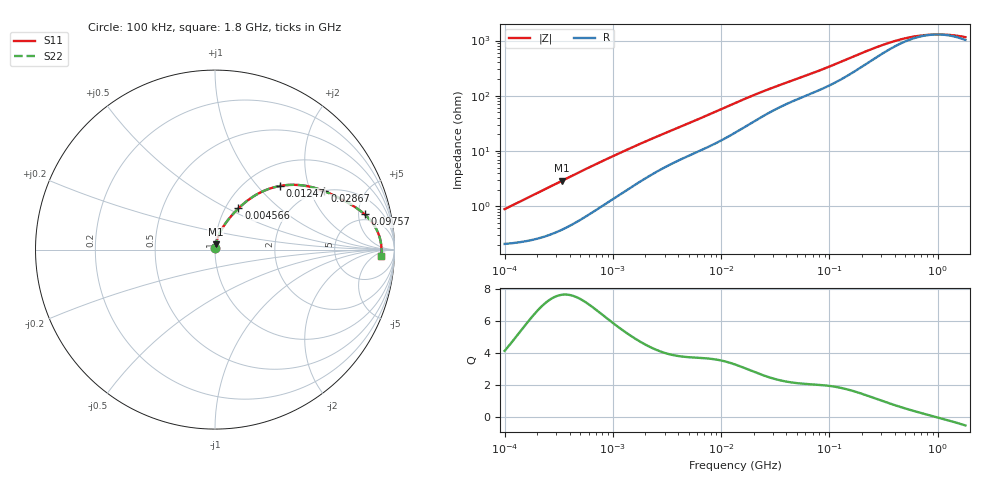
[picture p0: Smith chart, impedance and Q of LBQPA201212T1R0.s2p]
! LBQPA201212T1R0  S-PARAMETER MODEL  ( General Type )
! Model Generated by TAIYO YUDEN Corporation (http://www.ty-top.com)
! Version 1.0
! TAIYO YUDEN Control No. 191025NI43SB-FBB
! Copyright(c) 2019 TAIYO YUDEN CO.,LTD. All Rights Reserved.
! Product Description (link to TY-COMPAS)
! https://ds.yuden.co.jp/TYCOMPAS/or/detail?pn=LBQPA201212T1R0M&u=M
! Products Name : Inductors
! Characteristics :
!  Inductance : 1.0 uH , SRF(min) : 100 MHz , DC Resistance(max) : 0.247 Ohm
!  Rated Current : Saturation :700 mA , Temp Rise : 640 mA (20 degC)
!  Case Size : 2.0 x 1.25 / 0.079 x 0.049 [mm/inch] , Thickness : 1.25 / 0.049 [mm/inch]
!  (Conditions: Temperature = 25 degC , DC Bias Current/Voltage = 0A / 0V)
! External Node Assignments :
!  1  o---GGG---o  2
! GND o---------o GND
! Frequency Range : 0.1MHz  -  1800MHz  [ 402 STEP ]
# MHz S RI R 50
! Freq[MHz].  S11 Real  S11 Imag  S21 Real  S21 Imag  S12 Real  S12 Imag  S22 Real  S22 Imag
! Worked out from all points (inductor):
!   401 points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, 100 kHz to 1.8 GHz, reference 50 ohm
!   read as one part in series: L = 1.37 uH near 105 kHz
!   highest Q = 7.66 at 340.3 kHz (marker M1), where L = 1.35 uH
!   self-resonance near 976.1 MHz
!   S11 on the Smith chart (normalised r, x): 100 kHz: 1.00, +0.02; 4.566 MHz: 1.15, +0.57; 12.47 MHz: 1.39, +1.33; 28.67 MHz: 2.02, +2.52; 97.57 MHz: 4.00, +5.91; 1.8 GHz: 21, -11
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0.1  0.00214 0.00856  0.9979 -0.00856  0.9979 -0.00856  0.00214 0.00856
0.113029  0.00221 0.00967  0.9978 -0.00967  0.9978 -0.00967  0.00221 0.00967
0.340337  0.00457 0.0286  0.9954 -0.0286  0.9954 -0.0286  0.00457 0.0286
0.516129  0.00765 0.0425  0.9924 -0.0425  0.9924 -0.0425  0.00765 0.0425
1.246616  0.0263 0.0924  0.9737 -0.0924  0.9737 -0.0924  0.0263 0.0924
2.66389  0.0712 0.1635  0.9288 -0.1635  0.9288 -0.1635  0.0712 0.1635
4.566214  0.1308 0.2299  0.8692 -0.2299  0.8692 -0.2299  0.1308 0.2299
7.637621  0.2245 0.3027  0.7755 -0.3027  0.7755 -0.3027  0.2245 0.3027
12.46584  0.3604 0.3542  0.6396 -0.3542  0.6396 -0.3542  0.3604 0.3542
13.41641  0.3837 0.3579  0.6163 -0.3579  0.6163 -0.3579  0.3837 0.3579
18.90474  0.493 0.3569  0.507 -0.3569  0.507 -0.3569  0.493 0.3569
28.66948  0.6091 0.3256  0.3909 -0.3256  0.3909 -0.3256  0.6091 0.3256
42.42587  0.6949 0.286  0.3051 -0.286  0.3051 -0.286  0.6949 0.286
69.24595  0.7823 0.2357  0.2177 -0.2357  0.2177 -0.2357  0.7823 0.2357
97.57284  0.833 0.1971  0.167 -0.1971  0.167 -0.1971  0.833 0.1971
175.6488  0.8912 0.1278  0.1088 -0.1278  0.1088 -0.1278  0.8912 0.1278
266.3756  0.9117 0.0854  0.0883 -0.0854  0.0883 -0.0854  0.9117 0.0854
357.3983  0.9195 0.0609  0.0805 -0.0609  0.0805 -0.0609  0.9195 0.0609
542.0029  0.9252 0.0326  0.0748 -0.0326  0.0748 -0.0326  0.9252 0.0326
802.0705  0.9274 0.0104  0.0726 -0.0104  0.0726 -0.0104  0.9274 0.0104
1186.925  0.928 -0.0104  0.072 0.0104  0.072 0.0104  0.928 -0.0104
1800  0.9271 -0.0343  0.0729 0.0343  0.0729 0.0343  0.9271 -0.0343
